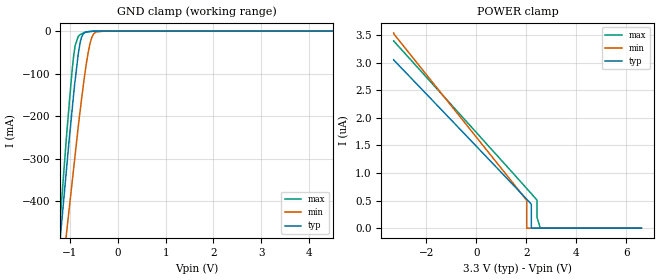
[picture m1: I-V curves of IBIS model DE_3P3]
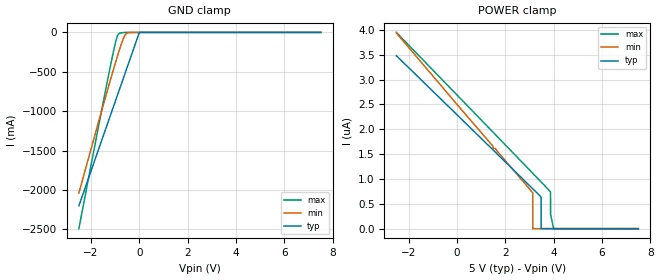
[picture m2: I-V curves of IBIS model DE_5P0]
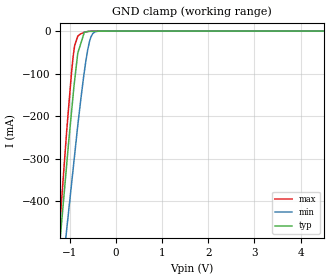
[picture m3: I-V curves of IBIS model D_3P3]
|Texas Instruments Incorporated
|THVD14xx 3.3-V to 5V RS-485 Transceivers With +/-16kV IEC ESD Protection
[IBIS Ver]   4.1
[File name]   thvd1452.ibs
[File Rev]   1.0
[Date]   01/25/2018
[Source]
| Texas Instruments Incorporated.
| Analog-eLab Design Center, HPA
| 12500 TI Blvd
| Dallas, TX -75243
[Notes]   Revision History:
| Rev 1.0: 01/25/2018
| - Initial version of the model
| - Model generated from simulations in SPECTRE
| - Warnings regarding combined Non-monotonicity of various models have been
|   reviewed and considered minor and can be ignored.
| - Model names with a trailing _3P3 contain the model for
|   3.3V operation. Model names with a trailing _5P0 contain the model
|   for 5.0V operation.
| - C_comp although listed in numerical order of value are
|   obtained from varying PVT conditions. For PVT conditions for
|   each specific value refer the buffer description under
|   respective [Model]. IBIS model user is responsible for using
|   appropriate C_comp to simulate for Signal Integrity.
[Disclaimer]
| This model is designed as an aid for customers of Texas Instruments.
| TI and its licensors and suppliers make no warranties, either expressed
| or implied, with respect to this  model, including the warranties of
| merchantability or fitness for a particular purpose. The model is
| provided solely on an "as is" basis. The entire risk as to its quality
| and performance is with the customer.
| This model is subject to change without notice. Texas Instruments
| Incorporated is not responsible for updating this model.
[Copyright]
(C) Copyright 2018 Texas Instruments Incorporated.All rights reserved.
|  Component THVD1452D 14-pin SOIC - D package
|  Part # THVD1452D
[Component]   THVD1452D
[Manufacturer]   TI
[Package]   |14 SOIC - D package
|   typ   min   max
R_pkg   0.1   0.08   0.12
L_pkg   1.0nH   0.8nH   1.2nH
C_pkg   0.2pF   0.16pF   0.24pF
[Pin]   signal_name   model_name   R_pin   L_pin   C_pin
1   NC   nc   NA   NA   NA
2   R   R_OUTPUT   NA   NA   NA
3   REB   REB_INPUT   NA   NA   NA
4   DE   DE_INPUT   NA   NA   NA
5   D   DE_INPUT   NA   NA   NA
6   GND   gnd   NA   NA   NA
7   GND   gnd   NA   NA   NA
8   NC   nc   NA   NA   NA
9   Y   Y_OUTPUT   NA   NA   NA
10   Z   Z_OUTPUT   NA   NA   NA
11   B   nc   NA   NA   NA
12   A   nc   NA   NA   NA
13   VCC   power   NA   NA   NA
14   VCC   power   NA   NA   NA
[Diff Pin]  inv_pin  vdiff  tdelay_typ tdelay_min tdelay_max
9   10   2   NA   NA   NA
|  Component THVD1452DGS 10-pin VSSOP - DGS package
|  Part # THVD1452DGS
[Component]   THVD1452DGS
[Manufacturer]   TI
[Package]   |14 VSSOP - DGS package
|   typ   min   max
R_pkg   0   0   0
L_pkg   0   0   0
C_pkg   0   0   0
[Pin]   signal_name   model_name   R_pin   L_pin   C_pin
1   R   R_OUTPUT   NA   NA   NA
2   REB   REB_INPUT   NA   NA   NA
3   DE   DE_INPUT   NA   NA   NA
4   D   D_INPUT   NA   NA   NA
5   GND   gnd   NA   NA   NA
6   Y   Y_OUTPUT   NA   NA   NA
7   Z   Z_OUTPUT   NA   NA   NA
8   B   nc   NA   NA   NA
9   A   nc   NA   NA   NA
10   VCC   power   NA   NA   NA
[Diff Pin]  inv_pin  vdiff  tdelay_typ tdelay_min tdelay_max
6   7   2   NA   NA   NA
|   Model Selectors
[Model Selector]   R_OUTPUT
R_3P3   3.3V   3-state
R_5P0   5V   3-state
[Model Selector]   D_INPUT
D_3P3   3.3V   Input
D_5P0   5V   Input
[Model Selector]   DE_INPUT
DE_3P3   3.3V   Input
DE_5P0   5V   Input
[Model Selector]   REB_INPUT
REB_3P3   3.3V   Input
REB_5P0   5V   Input
[Model Selector]   Y_OUTPUT
Y_3P3   3.3V   3-state
Y_5P0   5V   3-state
[Model Selector]   Z_OUTPUT
Z_3P3   3.3V   3-state
Z_5P0   5V   3-state
| Models and submodels in the file (12): DE_3P3 (Input), DE_5P0 (Input), D_3P3 (Input), D_5P0 (Input), REB_3P3 (Input), REB_5P0 (Input), R_3P3 (3-state), R_5P0 (3-state), Y_3P3 (3-state), Y_5P0 (3-state), Z_3P3 (3-state), Z_5P0 (3-state)
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|   DE_3P3 Model
[Model]   DE_3P3
Model_type   Input
Vinl = 0.462
Vinh = 0.7
|   typ   min   max
C_comp   5.008pF   4.849pF   5.22pF
|  Where Nom  PVT is Nominal Process,   3.3V,  25C
|   Fast PVT is Strong Process,   3.6V, -40C
|   Slow PVT is Weak Process,   3V, 150C
[Model spec]
|subparameter
Vinl   0.462   0.420   0.504
Vinh   2.211   2.010   2.412
[Voltage Range]   3.3   3   3.6
|Junction Temperature
[Temperature Range]   25   150   -40
[Power Clamp Reference]   3.3   3   3.6
[GND Clamp Reference]   0   0   0
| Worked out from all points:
|   GND clamp passes 1 mA (typ) near -0.61 V on its own axis
[GND Clamp]
|   Voltage   I(typ)   I(min)   I(max)
-3.3V     -3.278A    -2.936A    -3.779A
-1.238V   -530.9mA   -649.9mA   -491.4mA
-1.189V   -467.7mA   -596.9mA   -418.8mA
-1.068V   -317.4mA   -469.5mA   -239.1mA
-959.8mV  -189.7mA   -359.3mA   -96.7mA
-923.6mV  -148.3mA   -322.3mA   -58.46mA
-892.4mV  -115.4mA   -290.5mA   -33.91mA
-792.3mV  -29.54mA   -191.2mA   -8.958mA
-686.9mV  -3.242mA   -98.85mA   -2.881mA
-574.4mV  -556.7uA   -26.07mA   -1.159mA
-451.8mV  -177.9uA   -1.806mA   -57.26uA
6.6V      0A         0A         0A
[POWER Clamp]
|   Voltage   I(typ)   I(min)   I(max)
-3.3V     3.057uA    3.541uA    3.397uA
2.002V    532.4nA    511nA      727.1nA
2.016V    525.5nA    494.4nA    719.9nA
2.016V    525.4nA    429.1nA    719.7nA
2.016V    525.4nA    0A         719.7nA
2.201V    431.2nA    0A         626.1nA
2.201V    392.9nA    0A         625.9nA
2.201V    0A         0A         625.9nA
2.428V    0A         0A         501.2nA
2.429V    0A         0A         195.7nA
2.562V    0A         0A         0A
6.6V      0A         0A         0A
|   DE_5P5 Model
[Model]   DE_5P0
Model_type   Input
Vinl = 0.7
Vinh = 3.35
|   typ   min   max
C_comp   4.695pF   4.504pF   4.916pF
|  Where Nom  PVT is Nominal Process,   3.3V,  25C
|   Fast PVT is Strong Process,   3.6V, -40C
|   Slow PVT is Weak Process,   3V, 150C
[Model spec]
|subparameter
Vinl   0.462   0.420   0.504
Vinh   2.211   2.010   2.412
[Voltage Range]   5   4.5   5.5
|Junction Temperature
[Temperature Range]   25   150   -40
[Power Clamp Reference]   5   4.5   5.5
[GND Clamp Reference]   0   0   0
[GND Clamp]
|   Voltage   I(typ)   I(min)   I(max)
-2.5V     -2.201A    -2.039A    -2.491A
-1.759V   -1.549A    -1.216A    -1.307A
-1.185V   -1.043A    -591.8mA   -410.9mA
-1.054V   -928mA     -453.2mA   -220.1mA
-959.4mV  -844.5mA   -356.1mA   -96.19mA
-900mV    -792.3mA   -295.4mA   -38.98mA
-835.9mV  -735.8mA   -233.2mA   -13.46mA
-695.4mV  -612.1mA   -105.2mA   -3.342mA
-551.1mV  -485.1mA   -17.18mA   -490.8uA
-463.3mV  -407.8mA   -2.394mA   -412.6uA
-50.82uV  0A         0A         0A
7.5V      0A         0A         0A
[POWER Clamp]
|   Voltage   I(typ)   I(min)   I(max)
-2.5V     3.482uA    3.948uA    3.947uA
3.131V    804.3nA    720.8nA    1.116uA
3.135V    802.5nA    691.9nA    1.114uA
3.135V    802.4nA    573.1nA    1.114uA
3.135V    802.4nA    0A         1.114uA
3.48V     628.7nA    0A         939.5nA
3.481V    561.8nA    0A         939.2nA
3.481V    0A         0A         939.2nA
3.859V    0A         0A         745.7nA
3.871V    0A         0A         291.4nA
3.995V    0A         0A         0A
7.5V      0A         0A         0A
|   D_3P3 Model
[Model]   D_3P3
Model_type   Input
Vinl = 0.462
Vinh = 2.211
|   typ   min   max
C_comp   5.008pF   4.849pF   5.22pF
|  Where Nom  PVT is Nominal Process,   3.3V,  25C
|   Fast PVT is Strong Process,   3.6V, -40C
|   Slow PVT is Weak Process,   3V, 150C
[Model spec]
|subparameter
Vinl   0.462   0.420   0.504
Vinh   2.211   2.010   2.412
[Voltage Range]   3.3   3   3.6
|Junction Temperature
[Temperature Range]   25   150   -40
[Power Clamp Reference]   3.3   3   3.6
[GND Clamp Reference]   0   0   0
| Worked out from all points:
|   GND clamp passes 1 mA (typ) near -0.61 V on its own axis
[GND Clamp]
|   Voltage   I(typ)   I(min)   I(max)
-3.3V     -3.278A    -2.936A    -3.779A
-1.238V   -530.4mA   -649.5mA   -490.8mA
-1.189V   -467.6mA   -596.9mA   -418.7mA
-1.068V   -317.5mA   -469.6mA   -239.2mA
-923.8mV  -148.5mA   -322.6mA   -58.66mA
-892.5mV  -115.5mA   -290.6mA   -33.98mA
-825mV    -51.81mA   -221.8mA   -11.87mA
-686.9mV  -4.238mA   -98.87mA   -2.883mA
-611.5mV  -1.098mA   -45.16mA   -956uA
-556.5mV  -575.4uA   -19.03mA   -378.2uA
-389mV    -402.6uA   -378.7uA   -9.01uA
6.6V      0A         0A         0A
[POWER Clamp]
|   Voltage   I(typ)   I(min)   I(max)
-3.3V     0A         0A         0A
0V        0A         0A         0A
6.6V      0A         0A         0A
